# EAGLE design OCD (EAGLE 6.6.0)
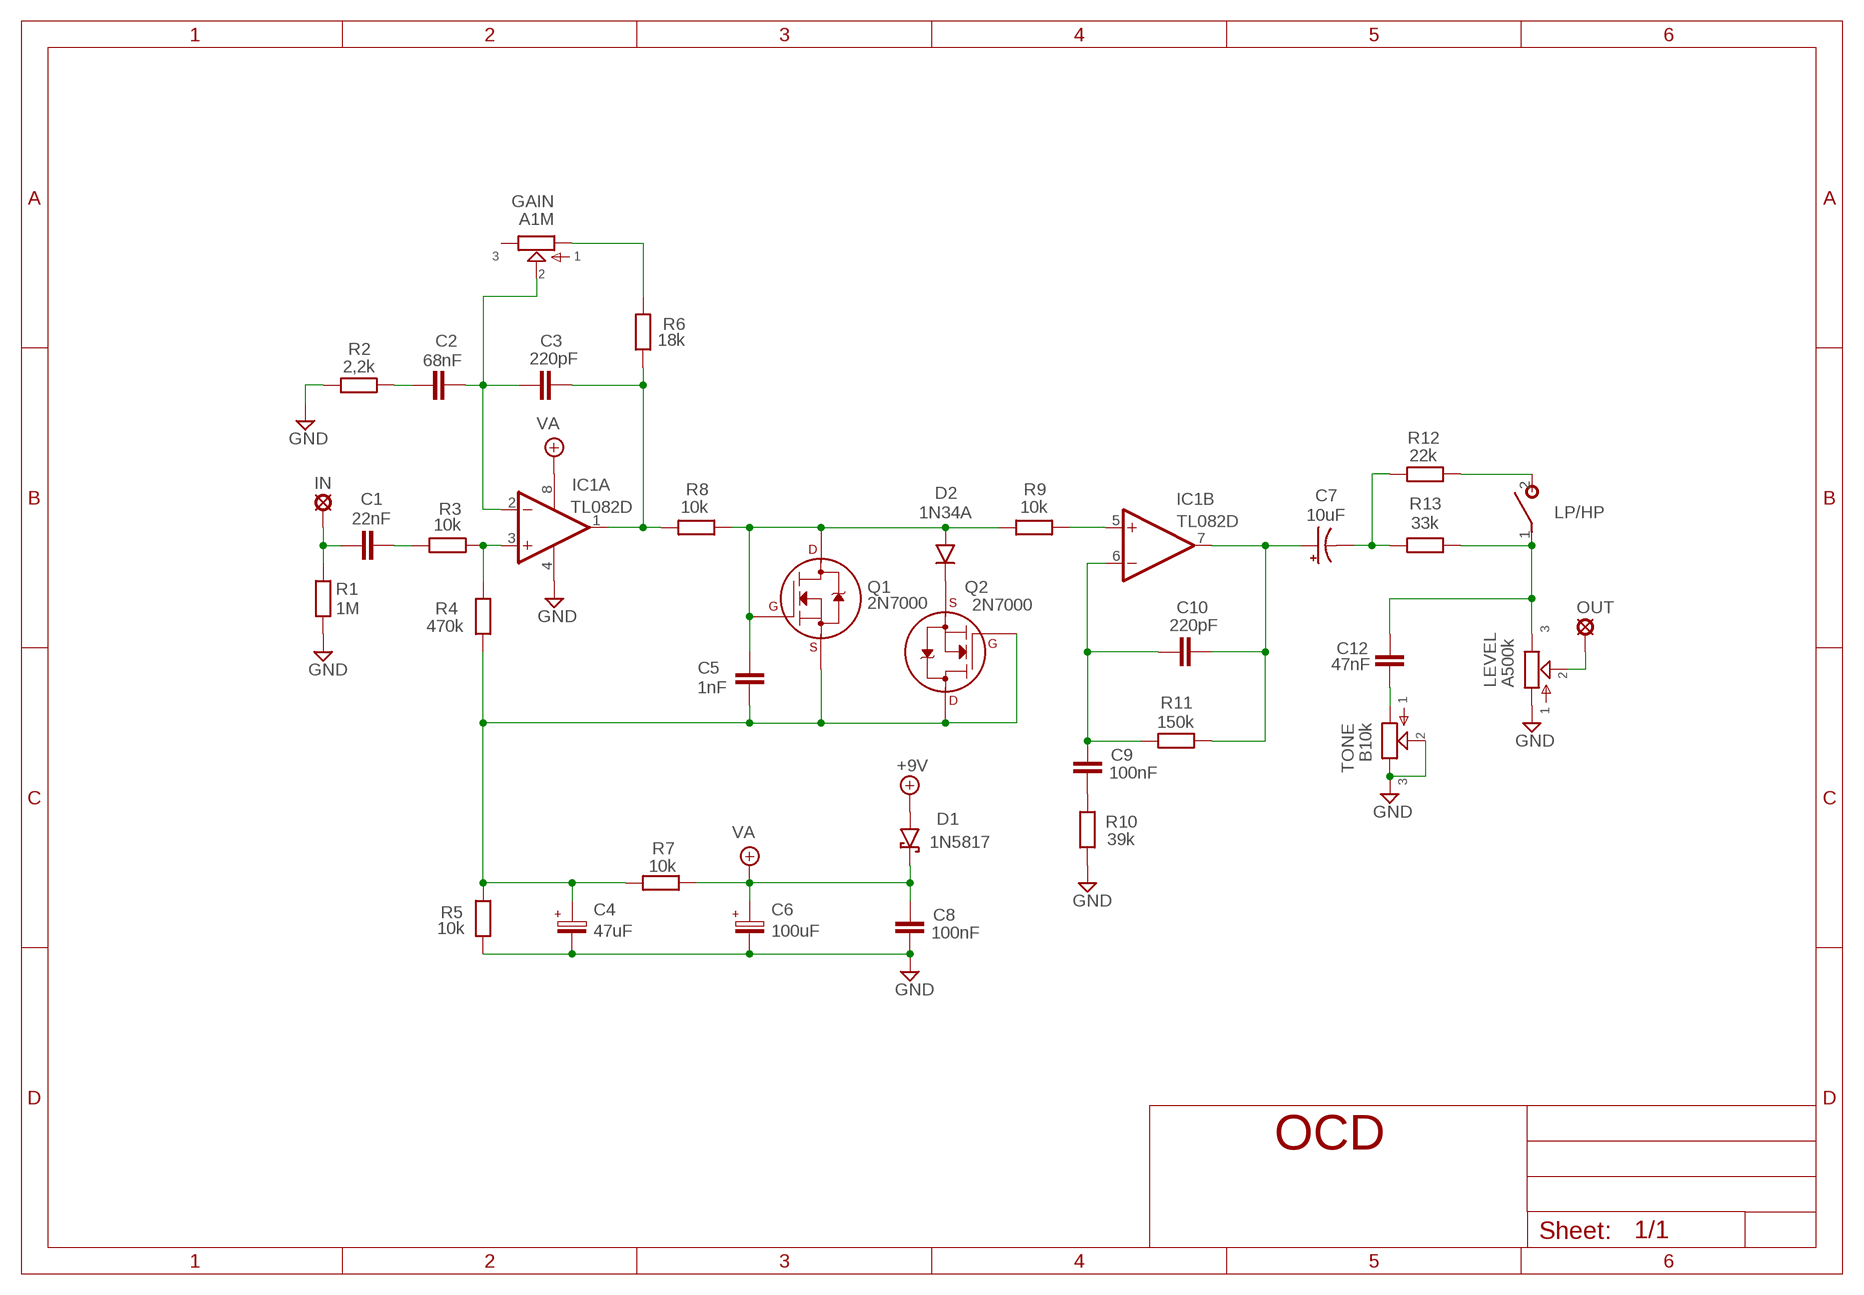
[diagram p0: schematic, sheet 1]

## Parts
+9V  +9V  +9V(T)1  [ROUND]
C1  22nF  22NF-82NF"  [4,5MM]
C2  68nF  22NF-82NF"  [4,5MM]
C3  220pF  050X030_0251  [050X030_025]
C4  47uF  063-EU  [063_025]
C5  1nF  1NF-15NF  [3,5MM]
C6  100uF  063-EU  [063_025]
C7  10uF  044A1  [044A]
C8  100nF  100NF-220NF  [7,5MM]
C9  100nF  100NF-220NF  [7,5MM]
C10  220pF  050X030_0251  [050X030_025]
C12  47nF  22NF-82NF"  [4,5MM]
D1  1N5817  [DO41-3]
D2  1N34A  DO07  [DO07]
GAIN  A1M  POT-EU16MM  [16MM]
GND  GND  GND(T)1  [ROUND]
GND4  GND  GND(T)1  [ROUND]
IC1  TL082D  [SO08]
IN  MCS10B  [MCS10B]
LEVEL  A500k  POT-EU16MM  [16MM]
LP/HP  SPST  [SPST]
OUT  MCS10B  [MCS10B]
Q1  2N7000  2N7000_TO92  [TO-92]
Q2  2N7000  2N7000_TO92  [TO-92]
R1  1M  6MM-EU3  [R0207/3]
R2  2,2k  6MM-EU3  [R0207/3]
R3  10k  6MM-EU3  [R0207/3]
R4  470k  6MM-EU3  [R0207/3]
R5  10k  6MM-EU3  [R0207/3]
R6  18k  6MM-EU3  [R0207/3]
R7  10k  6MM-EU3  [R0207/3]
R8  10k  6MM-EU3  [R0207/3]
R9  10k  6MM-EU3  [R0207/3]
R10  39k  6MM-EU3  [R0207/3]
R11  150k  6MM-EU3  [R0207/3]
R12  22k  6MM-EU3  [R0207/3]
R13  33k  6MM-EU3  [R0207/3]
TONE  B10k  POT-EU16MM  [16MM]

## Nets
+9V: +9V.1(+9V) D1.A
GND: C4.- C6.- C8.P$2 GND4.1(GND) GND.1(GND) IC1.4(P:V-) LEVEL.1 R1.1 R2.1 R5.1 R10.1 TONE.2 TONE.3
N$2: C3.2 IC1.1(A:OUT) R6.1 R8.1
N$3: C9.P$2 R10.2
N$4: D2.C Q2.1(S)
N$5: IC1.3(A:+IN) R3.2 R4.2
N$6: C4.+ C5.1 Q1.1(S) Q2.2(G) Q2.3(D) R4.1 R5.2 R7.1
N$7: C1.2 R3.1
N$8: C1.1 IN.MP R1.2
N$9: C5.2 D2.A Q1.2(G) Q1.3(D) R8.2 R9.1
N$10: C2.1 R2.2
N$11: C2.2 C3.1 GAIN.2 IC1.2(A:-IN)
N$12: IC1.5(B:+IN) R9.2
N$13: C7.1(+) C10.1 IC1.7(B:OUT) R11.2
N$14: C9.P$1 C10.2 IC1.6(B:-IN) R11.1
N$15: GAIN.1 R6.2
N$16: C7.2(-) R12.1 R13.1
N$17: LP/HP.2(S) R12.2
N$18: C12.1 LEVEL.3 LP/HP.1(P) R13.2
N$19: LEVEL.2 OUT.MP
N$20: C12.2 TONE.1
VA: C6.+ C8.P$1 D1.C IC1.8(P:V+) R7.2
Unconnected: GAIN.3

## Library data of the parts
+9V = gm-supply:+9V(T): +9V Voltage Supply
C1 C2 C12 = Mylar Kondensaattorit:22NF-82NF: 22nF-82nF
C3 C10 = Keraamiset kondensaattorit:050X030_025: 47 - 120pF
C4 C6 = Elektrolyytit:063-EU
C5 = Mylar Kondensaattorit:1NF-15NF: 1nF-15nF
C7 = gm-caps-tant:044A: .1 - 1.5µF
C8 C9 = Mylar Kondensaattorit:100NF-220NF: 100nF-220nF
D1 = Diodit:1N5817
D2 = Diodit:DO07: DO-07 Package
GAIN LEVEL TONE = gm-pots:POT-EU
GND GND4 = gm-supply:GND(T): Ground
IC1 = Operaatiovahvistimet:TL082: OP AMP
IN OUT = Padit:MCS10B: SOLDER PAD
LP/HP = Kytkimet:SPST
Q1 Q2 = transistors:2N700*: 2N7000, 2N7002, NDS7002A N-channel enhancement mode MOSFET
R1-R13 = Vastukset:6MM-EU: 6mm Resistors (European schematic symbol)

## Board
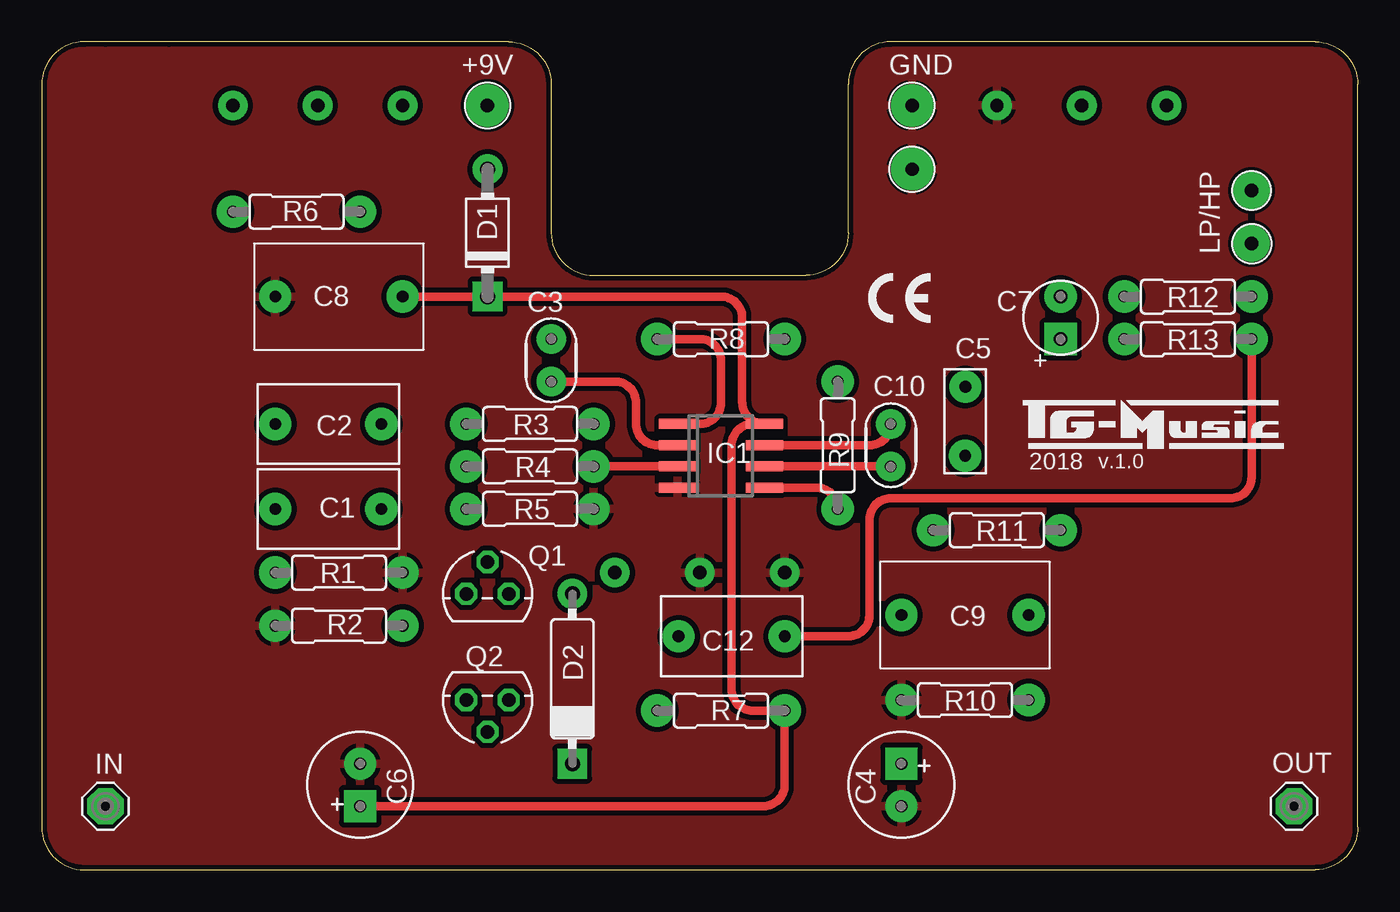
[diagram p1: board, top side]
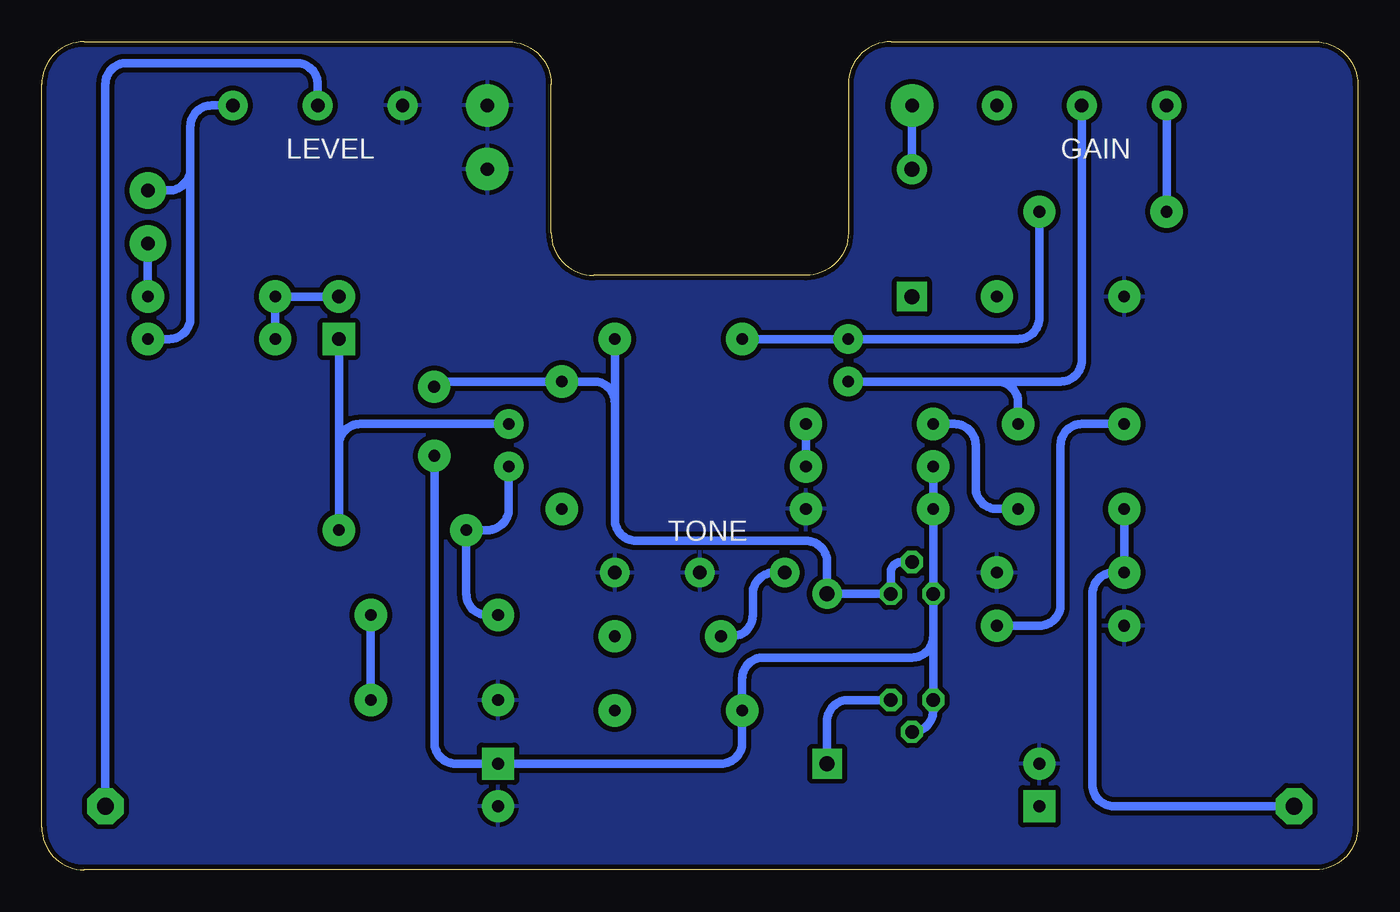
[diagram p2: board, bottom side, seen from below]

Size 78.74 x 49.53 mm. Coordinates in mm from the lower left corner, seen from the top.
Outline: 7.62,49.53 3.81,49.53
Outline: 78.74,2.54 78.74,46.99 arc90 76.2,49.53 50.8,49.53 arc90 48.26,46.99 48.26,38.1 arc-90 45.72,35.56 33.02,35.56 arc-90 30.48,38.1 30.48,46.99 arc90 27.94,49.53 2.54,49.53 arc90 0,46.99 0,2.54 arc90 2.54,0 76.2,0 arc90 78.74,2.54
Copper layers (1*16): Top 0.035mm / dielectric 1.5mm / Bottom 0.035mm
Design rules "ITEADstudio": minimum track width 10mil, minimum drill 12mil, track to track 12mil, track to pad 12mil, pad to pad 12mil, via to via 12mil, smd to smd 0mil, copper to edge 12mil, drill to drill 12mil, minimum pad ring 10mil, minimum via ring 6mil, stop-mask expansion 4mil, vias tented up to drill 100mil, thermal gap 10mil

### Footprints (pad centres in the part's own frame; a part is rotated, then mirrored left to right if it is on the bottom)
ROUND = drill 0.8 pad 2.54: 1 0,0
4,5MM = drill 0.7 pad 1.93: 1 -3.175,0; 2 3.175,0
050X030_025 = drill 0.7 pad 1.778: 1 -1.27,0; 2 1.27,0
063_025 = drill 0.7 pad 1.93 square: + -1.27,0 | drill 0.7 pad 1.93: - 1.27,0
3,5MM = drill 0.7 pad 1.93: 1 -1.905,0; 2 2.221,-0.016
044A = drill 0.8 pad 1.93 square: 1 -1.27,0 | drill 0.8 pad 1.93: 2 1.27,0
7,5MM = drill 0.7 pad 1.93: P$1 -3.81,0; P$2 3.81,0
DO41-3 = drill 0.9 pad 1.778: A 3.81,0 | drill 0.9 pad 1.778 square: C -3.81,0
DO07 = drill 0.9 pad 1.778: A 5.08,0 | drill 0.9 pad 1.778 square: C -5.08,0
16MM = drill 0.8 pad 1.778: 1 5.08,0; 2 0,0; 3 -5.08,0
SO08 = smd 0.6 x 2.2: 1 -1.905,-2.6; 2 -0.635,-2.6; 3 0.635,-2.6; 4 1.905,-2.6; 5 1.905,2.6; 6 0.635,2.6; 7 -0.635,2.6; 8 -1.905,2.6
MCS10B = drill 1.016 pad 2.159 octagon: MP 0,0
SPST = drill 0.8 pad 2.184: 1 -1.27,0; 2 1.905,0
TO-92 = drill 0.813 octagon: 1 -1.27,0; 2 0,1.905; 3 1.27,0
R0207/3 = drill 0.7 pad 1.93: 1 -3.81,0; 2 3.81,0

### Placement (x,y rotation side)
+9V  26.67,45.72 0 top
C1  17.14,21.59 0 top
C2  17.14,26.67 0 top
C3  30.48,30.48 90 top
C4  51.44,5.08 270 top
C5  55.24,26.67 90 top
C6  19.05,5.08 90 top
C7  60.96,33.02 90 top
C8  17.78,34.29 180 top
C9  55.24,15.24 0 top
C10  50.8,25.4 270 top
C12  41.27,13.97 180 top
D1  26.67,38.1 90 top
D2  31.75,11.43 90 top
GAIN  16.51,45.72 0 bottom
GND  52.07,45.72 0 top
GND4  52.07,41.91 0 top
IC1  40.64,24.77 270 top
IN  3.81,3.81 0 top
LEVEL  62.23,45.72 0 bottom
LP/HP  72.39,39.37 270 top
OUT  74.93,3.81 0 top
Q1  26.67,16.51 0 top
Q2  26.67,10.16 180 top
R1  17.78,17.78 180 top
R2  17.78,14.61 0 top
R3  29.21,26.67 0 top
R4  29.21,24.13 0 top
R5  29.21,21.59 180 top
R6  15.24,39.37 180 top
R7  40.64,9.53 0 top
R8  40.64,31.75 0 top
R9  47.62,25.4 270 top
R10  55.24,10.16 0 top
R11  57.15,20.32 0 top
R12  68.58,34.29 0 top
R13  68.58,31.75 0 top
TONE  39.37,17.78 0 bottom

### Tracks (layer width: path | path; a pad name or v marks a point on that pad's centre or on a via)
+9V
  Bottom 0.508: +9V.1 D1.A
GND
  pour Bottom: 0,2.54 0,46.99 arc-90 2.54,49.53 27.94,49.53 arc-90 30.48,46.99 30.48,38.1 arc90 33.02,35.56 45.72,35.56 arc90 48.26,38.1 48.26,46.99 arc-90 50.8,49.53 76.2,49.53 arc-90 78.74,46.99 78.74,2.54 arc-90 76.2,0 2.54,0 arc-90
  pour Top: 0,2.54 0,46.99 arc-90 2.54,49.53 27.94,49.53 arc-90 30.48,46.99 30.48,38.1 arc90 33.02,35.56 45.72,35.56 arc90 48.26,38.1 48.26,46.99 arc-90 50.8,49.53 76.2,49.53 arc-90 78.74,46.99 78.74,2.54 arc-90 76.2,0 2.54,0 arc-90
N$2
  Top 0.508: IC1.1 39.37,26.67 arc90 40.64,27.94 40.64,30.48 arc90 39.37,31.75 R8.1
  Bottom 0.508: R8.1 C3.2 20.32,31.75 arc-90 19.05,33.02 R6.1
N$3
  Bottom 0.508: C9.P$2 R10.2
N$4
  Bottom 0.508: Q2.1 30.48,10.16 arc-90 31.75,8.89 D2.C
N$5
  Top 0.508: IC1.3 R4.2
  Bottom 0.508: R4.2 R3.2
N$6
  Bottom 0.508: R4.1 R5.2 Q1.1 25.4,13.97 | 25.4,13.97 Q2.3 25.4,9.53 arc90 Q2.2 | 25.4,13.97 arc90 26.67,12.7 35.56,12.7 arc-90 36.83,11.43 R7.1 36.83,7.62 arc90 38.1,6.35 C4.+ 53.98,6.35 arc90 55.24,7.62 C5.1
N$7
  Bottom 0.508: R3.1 24.13,26.67 arc90 22.86,25.4 22.86,22.86 arc-90 21.59,21.59 C1.2
N$8
  Bottom 0.508: IN.MP 14.61,3.81 arc90 15.88,5.08 15.88,16.51 arc90 14.61,17.78 R1.2 C1.1
N$9
  Bottom 0.508: Q1.2 27.3,18.41 arc-90 27.94,17.78 Q1.3 D2.A 31.75,18.41 arc-90 33.02,19.68 43.18,19.68 arc90 44.45,20.95 44.45,27.94 | 44.45,27.94 R8.2 | 44.45,27.94 arc-90 45.72,29.21 R9.1 54.94,29.21 arc-90 C5.2
N$10
  Bottom 0.508: C2.1 16.51,26.67 arc-90 17.78,25.4 17.78,15.88 arc90 19.05,14.61 R2.2
N$11
  Top 0.508: C3.1 34.29,29.21 arc-90 35.56,27.94 35.56,26.67 arc90 36.83,25.4 IC1.2
  Bottom 0.508: C3.1 21.59,29.21 | 21.59,29.21 17.78,29.21 arc-90 16.51,30.48 GAIN.2 | C2.2 20.32,27.94 arc-90 21.59,29.21
N$12
  Top 0.508: IC1.5 46.35,22.86 arc-90 R9.2
N$13
  Top 0.508: IC1.7 49.53,25.4 arc90 C10.1
  Bottom 0.508: C7.1 60.96,25.4 | 60.96,25.4 R11.2 | C10.1 59.69,26.67 arc-90 60.96,25.4
N$14
  Top 0.508: IC1.6 C10.2
  Bottom 0.508: C10.2 50.8,21.59 arc90 52.07,20.32 R11.1 53.34,16.51 arc-90 52.07,15.24 C9.P$1
N$15
  Bottom 0.508: GAIN.1 R6.2
N$16
  Bottom 0.508: C7.2 R12.1 R13.1
N$17
  Bottom 0.508: LP/HP.2 R12.2
N$18
  Top 0.508: C12.1 48.26,13.97 arc90 49.53,15.24 49.53,20.95 arc-90 50.8,22.23 71.12,22.23 arc90 72.39,23.5 R13.2
  Bottom 0.508: 69.85,41.91 69.85,44.45 arc90 68.58,45.72 LEVEL.3 | 69.85,41.91 69.85,33.02 arc90 71.12,31.75 R13.2 | LP/HP.1 71.12,40.64 arc-90 69.85,41.91
N$19
  Bottom 0.508: OUT.MP 74.93,46.99 arc90 73.66,48.26 63.5,48.26 arc90 62.23,46.99 LEVEL.2
N$20
  Bottom 0.508: TONE.1 34.92,17.78 arc-90 36.2,16.51 36.2,15.24 arc90 37.47,13.97 C12.2
VA
  Top 0.508: C8.P$1 D1.C 40.64,34.29 arc-90 41.91,33.02 41.91,28 arc90 IC1.8 42.55,26.67 arc90 41.27,25.4 41.27,10.79 arc90 42.55,9.53 R7.2 44.45,5.08 arc-90 43.18,3.81 C6.+
  Bottom 0.508: R7.2 43.81,9.53

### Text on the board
tNames: 2018 | v.1.0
